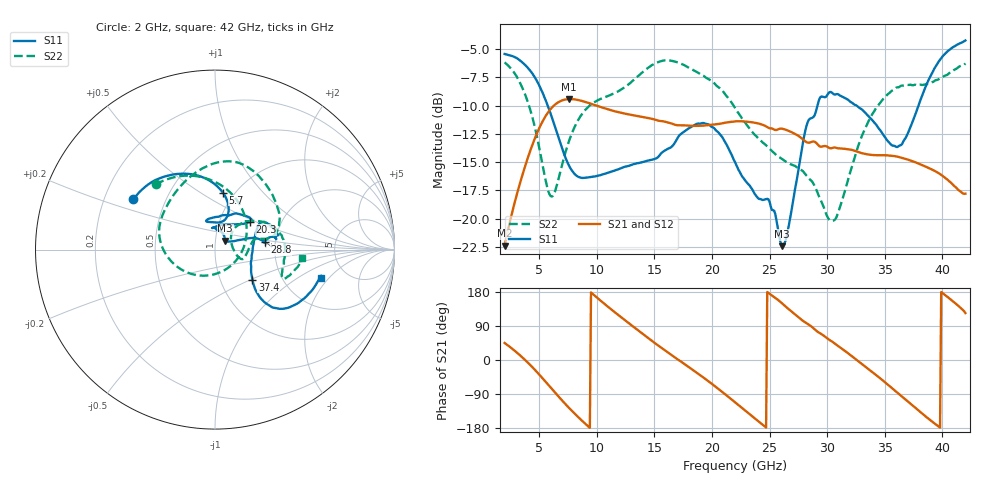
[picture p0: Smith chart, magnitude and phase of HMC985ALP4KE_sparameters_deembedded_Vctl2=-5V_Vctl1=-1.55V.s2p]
!s2p File: Measurements: S11, S21, S12, S22
# GHz S dB R 50.0
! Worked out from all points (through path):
!   401 points, 2 GHz to 42 GHz, reference 50 ohm
!   highest |S21| = -9.43 dB at 7.6 GHz (marker M1); lowest = -22.4 dB at 2 GHz (marker M2)
!   lowest |S11| = -22.4 dB at 26.1 GHz (marker M3), VSWR 1.16, Z = 55.8 + j5.55 ohm
!   |S11| at or under -10 dB: 5.739 GHz to 29.16 GHz (23.42 GHz wide, 134 % of centre); 32.54 GHz to 37.93 GHz (5.392 GHz wide, 15.3 % of centre)
!   |S22| runs from -20.2 to -6.0 dB; largest |S21 - S12| = 0.00035
!   S11 on the Smith chart (normalised r, x): 2 GHz: 0.33, +0.25; 5.7 GHz: 0.88, +0.63; 20.3 GHz: 1.39, +0.46; 28.8 GHz: 1.76, +0.17; 37.4 GHz: 1.42, -0.51; 42 GHz: 3.28, -1.64
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2  -5.44 148.5  -22.41 44.9  -22.42 44.9  -6.18 132.3
3.6  -6.24 122.1  -15.96 5.2  -15.97 5.2  -8.58 88.5
4.7  -7.64 101.1  -12.72 -28.2  -12.72 -28.2  -12.25 46.4
5.7  -9.89 82.1  -10.72 -62.3  -10.72 -62.2  -17.25 -19.0
6.3  -11.65 73.7  -9.99 -83.2  -9.99 -83.2  -17.80 -75.6
7.6  -15.34 72.4  -9.43 -126.6  -9.44 -126.6  -13.11 -150.9
8.7  -16.40 85.5  -9.59 -159.7  -9.60 -159.7  -10.78 179.6
12.1  -15.55 107.2  -10.64 113.2  -10.64 113.2  -8.60 132.4
15.4  -14.47 81.5  -11.35 36.8  -11.36 36.8  -6.13 84.2
17.8  -12.15 51.5  -11.77 -14.6  -11.77 -14.6  -6.55 56.5
20.3  -12.14 38.4  -11.66 -70.2  -11.67 -70.2  -8.14 23.7
22  -15.01 52.4  -11.41 -111.6  -11.41 -111.6  -10.21 12.0
24.4  -18.36 97.7  -11.71 -170.9  -11.71 -170.9  -13.27 13.2
26.1  -22.44 41.0  -12.05 149.0  -12.06 149.0  -14.75 -2.8
28.7  -11.09 7.8  -13.20 86.8  -13.21 86.9  -16.74 -18.8
28.8  -11.03 8.9  -13.18 84.3  -13.19 84.3  -16.90 -18.4
30.7  -9.03 15.3  -13.72 42.4  -13.72 42.5  -20.07 25.6
33.2  -10.54 30.6  -14.26 -14.6  -14.27 -14.6  -12.26 40.6
35.4  -13.29 8.1  -14.42 -68.4  -14.43 -68.4  -8.90 18.5
37.4  -11.47 -38.7  -14.93 -120.0  -14.93 -120.0  -8.21 -3.5
39.7  -6.09 -41.7  -16.00 -176.2  -16.00 -176.1  -7.66 -23.1
42  -4.25 -14.8  -17.80 123.9  -17.80 124.0  -6.28 -5.7
